(* Logix 5000 AddOnInstructionDefinition export Banner_Q20EAF_Param_v4; software revision 33.00 *)

TYPE Banner_IOL_Port_v4 :   // UDT that has all of the data items necessary to communicate with a specific Port on a IO-Link Master
STRUCT
   Port_Controlled : INT;   // Each bit represents a port on an IO-Link Master. Set to 1 to tell AOI to control that port.
   Port_Activate : INT;   // Each bit represents a port on an IO-Link Master. When ON that port will process any commands in queue.
   Port_Read : INT;   // Each bit represents a port on an IO-Link Master. Used to determine when device AOI has requested a Read command.
   Port_Write : INT;   // Each bit represents a port on an IO-Link Master. Used to determine when device AOI has requested a Write command.
   Port_RW_Complete : INT;   // Each bit represents a port on an IO-Link Master. Tells device AOI that Read or Write request has been completed.
   Port_Device_Read : INT;
   Data_Transfer : SINT[190];   // Array to transfer data from IO-Master to device AOIs.
END_STRUCT
END_TYPE

TYPE Banner_Q20EAF_RD_v4 :   // UDT that stores the Write Data for a Q20 EAF.
STRUCT
   Master_Cycle_Time : INT;
   Min_Cycle_Time : INT;
   M_Sequence_Capability : INT;
   IO_Link_Version_ID : INT;
   Process_Data_Input_Length : INT;
   Process_Data_Output_Length : INT;
   Combined_Vendor_ID : DINT;   // IO-Link Vendor ID
   Vendor_ID1 : INT;
   Vendor_ID2 : INT;
   Combined_Device_ID : DINT;   // IO-Link Device ID
   Device_ID1 : INT;
   Device_ID2 : INT;
   Device_ID3 : INT;
   Serial_Number : STRING;
   Teach_State : INT;   // 0 = Idle, 1 = SP1 Success, 4 = Wait for Command, 5 = Busy, 7 = Error.
   SP1_TP1 : SINT;
   SP1_TP2 : SINT;
   Current_Setpoint : DINT;   // Current setpoint selected by either the POT or SP1.
   All_Time_Run_Time : DINT;   // Read only counter that tracks the total time sensor has been running since manufacture. Value in Hours.
   Taught_Distance_Status : INT;   // 0 = Not taught, 1 = Taught, 2 = Coerced to near limit, 3 = Coerced to far limit.
END_STRUCT
END_TYPE

TYPE Banner_Q20EAF_v4 :   // All of the parameters for a Q20 EAF.
STRUCT
   Initial_Global_Read : BOOL;   // Determines if all of the IO-Link data has been read into the PLC yet
   Command : INT;   // Value placed in here will activate a read or write to a specifc IO-Link Index
   Read_Data : Banner_Q20EAF_RD_v4;   // Read Only Data
   Write_Data : Banner_Q20EAF_WD_v4;   // Write Data
   Archive : Banner_Q20EAF_WD_v4;   // Archive Data
   Reset : BOOL;   // Resets AOI. This will force a complete parameter read of the sensor.
END_STRUCT
END_TYPE

TYPE Banner_Q20EAF_WD_v4 :   // UDT that stores the Write Data for a Q20 EAF.
STRUCT
   System_Command : INT;   // See IODD file for list of commands that can be activated via the System Command interface
   Parameter_Access_Lock : SINT;   // Write access to all parameters is prohibited while value is 1. Only this parameter can be adjusted when value is 1.
   Data_Storage_Lock : SINT;   // Automatic data storage is disabled when this value is equal to 1. Read access is not affected.
   Local_Parameterization_Lock : SINT;   // Parameterization via local control elements on device is disabled.
   Local_User_Interface_Lock : SINT;   // Operation of local user interface is disabled.
   BDC1_Setpoint_SP1 : DINT;
   BDC1_Setpoint_SP2 : DINT;
   BDC1_Swithpoint_Logic : INT;   // 0 = Light Operate, 1 = Dark Operate
   BDC1_BDC_Mode : INT;   // 1 = 1-Pt BGS, 128 = 2-Pt, 129 = Dynamic, 130 = Window or FGS, 131 = Dual
   BDC1_Hysteresis : DINT;   // Should always be 0
   BDC1_Setpoint_Selection : SINT;   // 0 = Local (POT), 1 = Remote (AOI).
   Delay_Mode : INT;   // 0=Disabled, 1=On Off Delay, 2=Oneshot
   Delay_Timer_1 : DINT;   // 0 to 90000 ms
   Delay_Timer_2 : DINT;   // 0 to 90000 ms
   Teach_Offset_mode : INT;   // 0 = Auto, 1 = User Controlled.
   User_Teach_Offset : DINT;   // User selected teach offset.
   Resettable_Run_Time : DINT;
   All_Time_Run_Time_Event_Time : DINT;
   Resettable_Run_Time_Event_Time : DINT;
   Pin_2_Configuration : SINT;   // 0 = Detection Output, 1 = Complimentary Output.
   Response_Speed : SINT;   // 0 = High Speed (450 microsecs), 1 = Cross-talk Only (1.1 ms), 2 = Robust (1.7 ms ON, 1.1 ms OFF).
END_STRUCT
END_TYPE

ADD_ON_INSTRUCTION Banner_Q20EAF_Param_v4   (* revision 4.0, vendor Banner Engineering *)
// AOI to read and write parameter data to an IO-Link Q20 EAF.
VAR_IN_OUT
   Q20 : Banner_Q20EAF_v4; {required}
   Port_Data : Banner_IOL_Port_v4; {required}
END_VAR
VAR_INPUT
   Port : DINT; {required}
END_VAR
VAR
   Local_Control : DINT; {access None}
   Global_Read_Command_Value : INT; {access None}
   Global_Write_Command_Value : INT; {access None}
   Command_Being_Processed : BOOL; {access None}
   Update_Archive : BOOL; {access None}
   Index_Write_Inprocess : INT; {access None}
   Index_Write_Control : INT; {access None}
   Inprocess_Index : DINT; {access None}
END_VAR

ROUTINE Logic   (* ladder *)
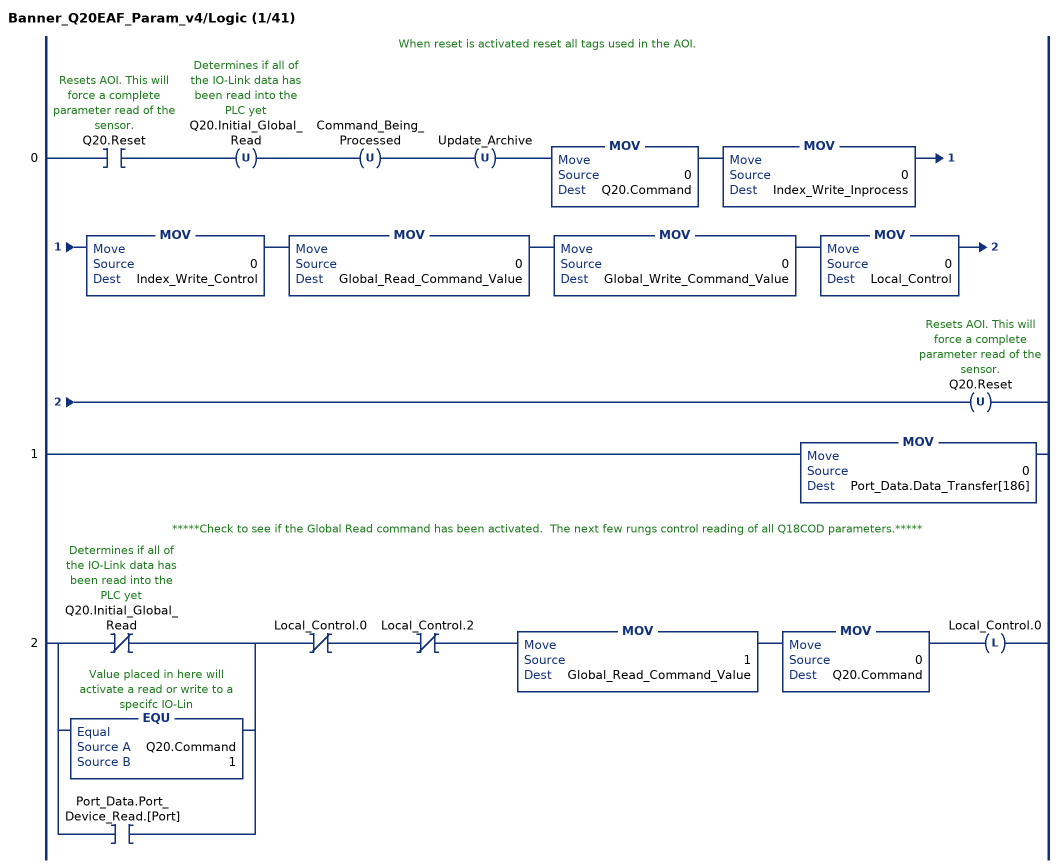
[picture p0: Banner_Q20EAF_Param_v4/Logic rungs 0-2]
   // When reset is activated reset all tags used in the AOI.
   0: XIC(Q20.Reset)OTU(Q20.Initial_Global_Read)OTU(Command_Being_Processed)OTU(Update_Archive)MOV(0,Q20.Command)MOV(0,Index_Write_Inprocess)MOV(0,Index_Write_Control)MOV(0,Global_Read_Command_Value)MOV(0,Global_Write_Command_Value)MOV(0,Local_Control)OTU(Q20.Reset);
   1: MOV(0,Port_Data.Data_Transfer[186]);
   // *****Check to see if the Global Read command has been activated.  The next few rungs control reading of all Q18COD parameters.*****
   2: [XIO(Q20.Initial_Global_Read) ,EQU(Q20.Command,1) ,XIC(Port_Data.Port_Device_Read.[Port]) ]XIO(Local_Control.0)XIO(Local_Control.2)MOV(1,Global_Read_Command_Value)MOV(0,Q20.Command)OTL(Local_Control.0);
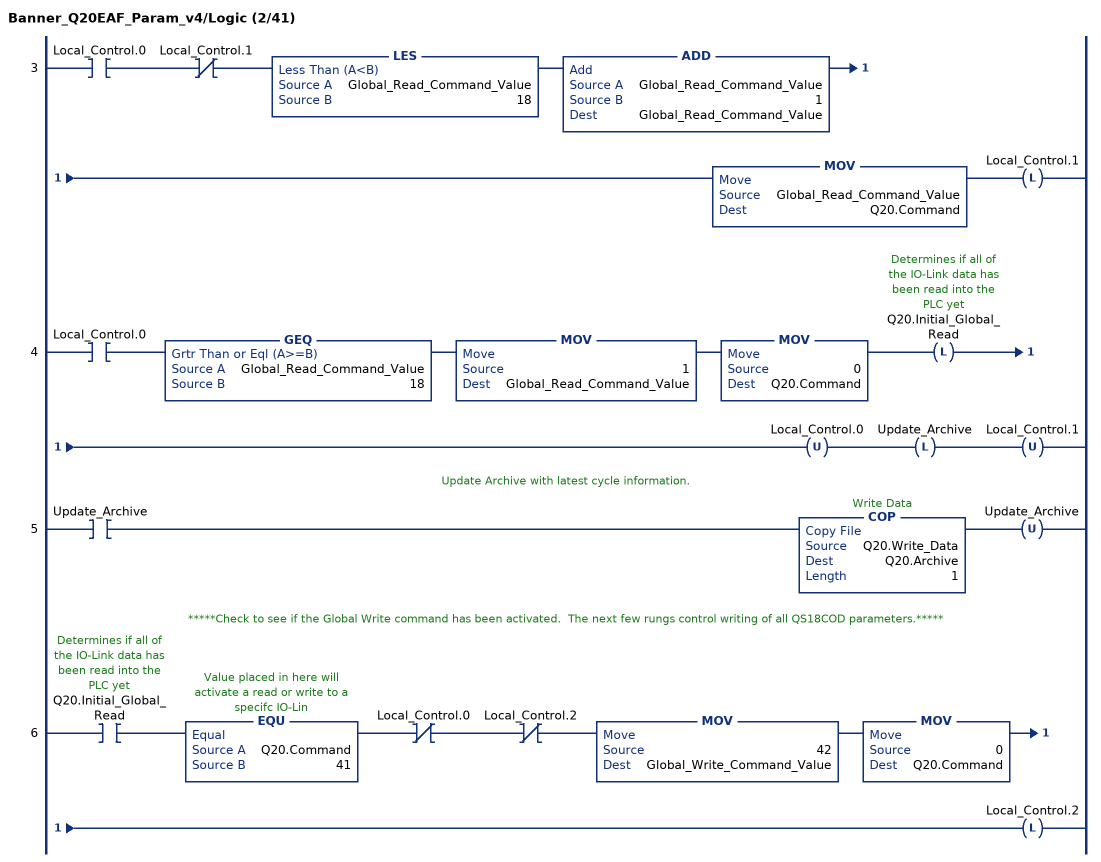
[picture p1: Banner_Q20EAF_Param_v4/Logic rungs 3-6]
   3: XIC(Local_Control.0)XIO(Local_Control.1)LES(Global_Read_Command_Value,18)ADD(Global_Read_Command_Value,1,Global_Read_Command_Value)MOV(Global_Read_Command_Value,Q20.Command)OTL(Local_Control.1);
   4: XIC(Local_Control.0)GEQ(Global_Read_Command_Value,18)MOV(1,Global_Read_Command_Value)MOV(0,Q20.Command)OTL(Q20.Initial_Global_Read)OTU(Local_Control.0)OTL(Update_Archive)OTU(Local_Control.1);
   // Update Archive with latest cycle information.
   5: XIC(Update_Archive)COP(Q20.Write_Data,Q20.Archive,1)OTU(Update_Archive);
   // *****Check to see if the Global Write command has been activated.  The next few rungs control writing of all QS18COD parameters.*****
   6: XIC(Q20.Initial_Global_Read)EQU(Q20.Command,41)XIO(Local_Control.0)XIO(Local_Control.2)MOV(42,Global_Write_Command_Value)MOV(0,Q20.Command)OTL(Local_Control.2);
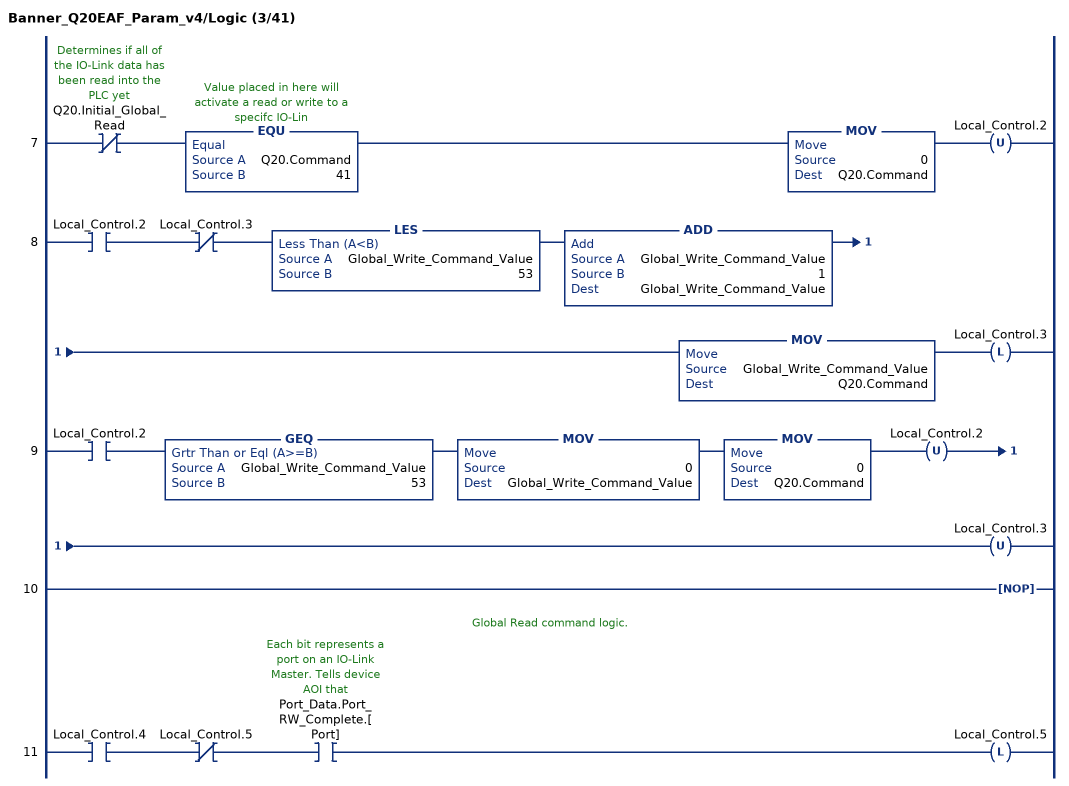
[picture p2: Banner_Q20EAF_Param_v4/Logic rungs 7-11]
   7: XIO(Q20.Initial_Global_Read)EQU(Q20.Command,41)MOV(0,Q20.Command)OTU(Local_Control.2);
   8: XIC(Local_Control.2)XIO(Local_Control.3)LES(Global_Write_Command_Value,53)ADD(Global_Write_Command_Value,1,Global_Write_Command_Value)MOV(Global_Write_Command_Value,Q20.Command)OTL(Local_Control.3);
   9: XIC(Local_Control.2)GEQ(Global_Write_Command_Value,53)MOV(0,Global_Write_Command_Value)MOV(0,Q20.Command)OTU(Local_Control.2)OTU(Local_Control.3);
   10: NOP();
   // Global Read command logic.
   11: XIC(Local_Control.4)XIO(Local_Control.5)XIC(Port_Data.Port_RW_Complete.[Port])OTL(Local_Control.5);
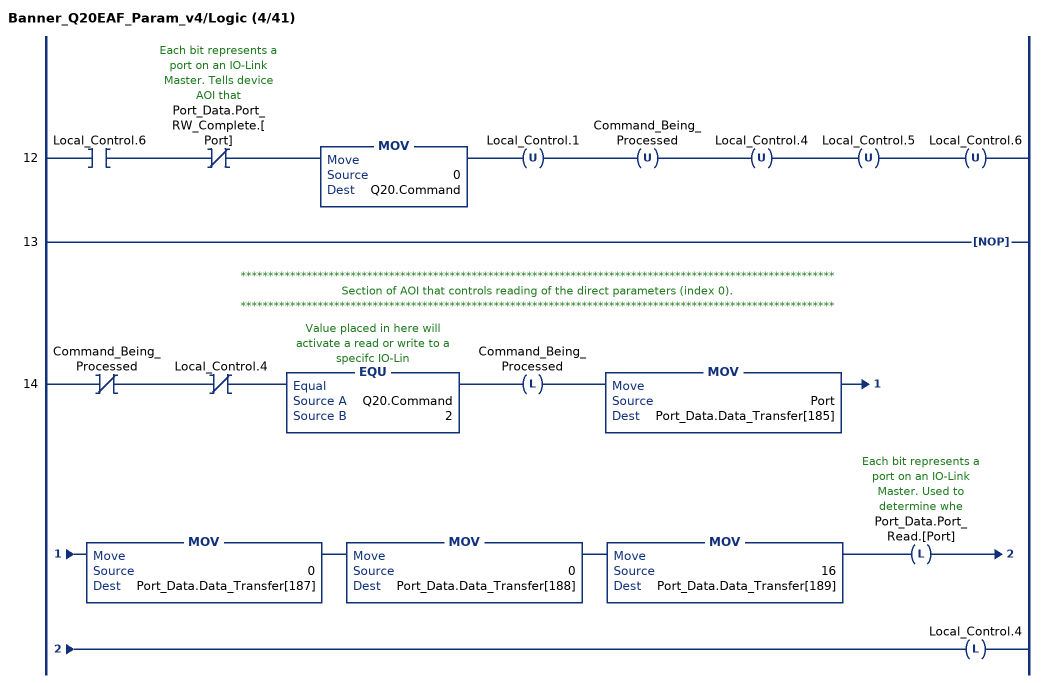
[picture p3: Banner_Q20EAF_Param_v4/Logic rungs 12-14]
   12: XIC(Local_Control.6)XIO(Port_Data.Port_RW_Complete.[Port])MOV(0,Q20.Command)OTU(Local_Control.1)OTU(Command_Being_Processed)OTU(Local_Control.4)OTU(Local_Control.5)OTU(Local_Control.6);
   13: NOP();
   // ************************************************************************************************************
   // Section of AOI that controls reading of the direct parameters (index 0).
   // ************************************************************************************************************
   14: XIO(Command_Being_Processed)XIO(Local_Control.4)EQU(Q20.Command,2)OTL(Command_Being_Processed)MOV(Port,Port_Data.Data_Transfer[185])MOV(0,Port_Data.Data_Transfer[187])MOV(0,Port_Data.Data_Transfer[188])MOV(16,Port_Data.Data_Transfer[189])OTL(Port_Data.Port_Read.[Port])OTL(Local_Control.4);
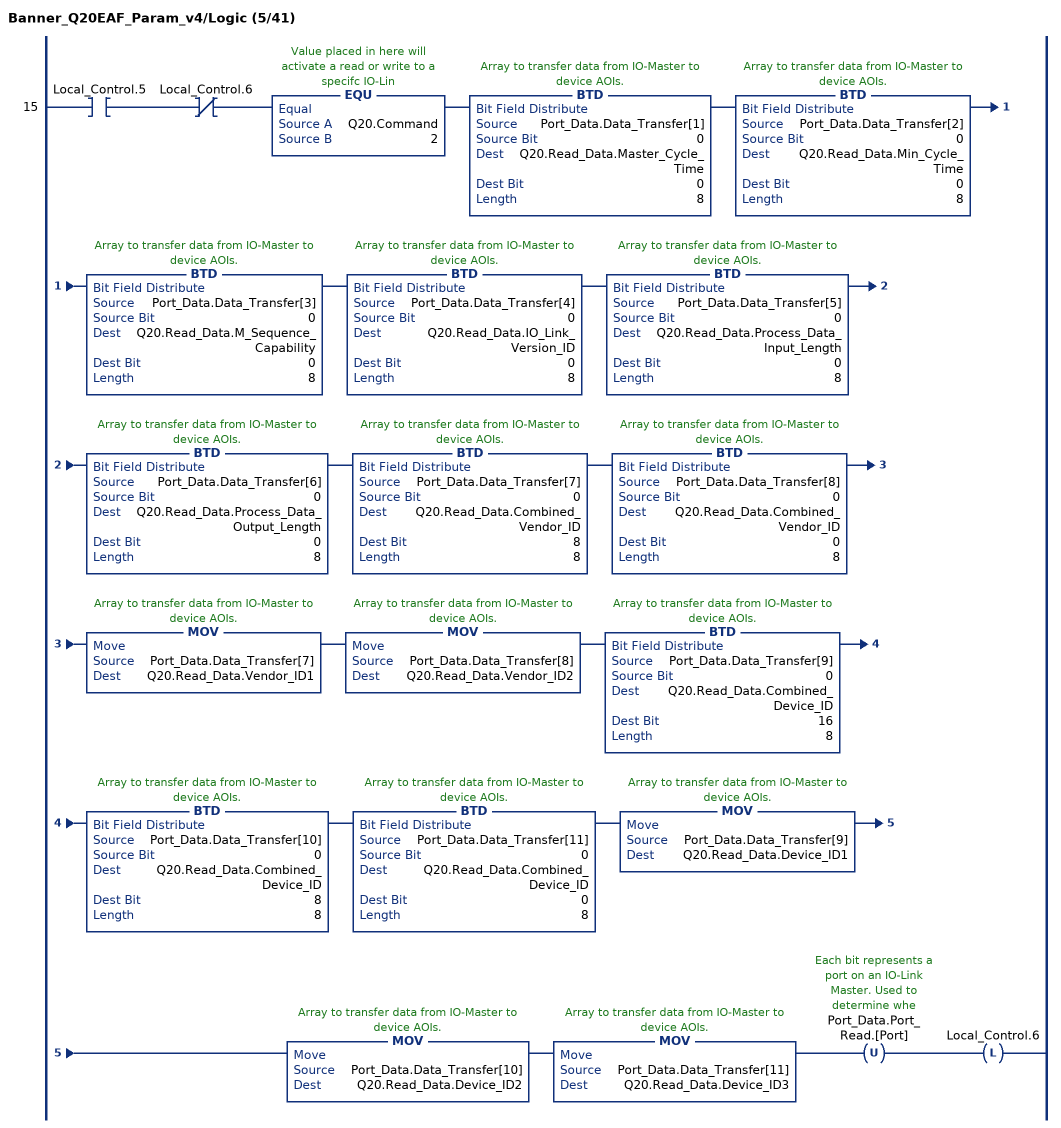
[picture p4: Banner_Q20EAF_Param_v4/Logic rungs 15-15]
   15: XIC(Local_Control.5)XIO(Local_Control.6)EQU(Q20.Command,2)BTD(Port_Data.Data_Transfer[1],0,Q20.Read_Data.Master_Cycle_Time,0,8)BTD(Port_Data.Data_Transfer[2],0,Q20.Read_Data.Min_Cycle_Time,0,8)BTD(Port_Data.Data_Transfer[3],0,Q20.Read_Data.M_Sequence_Capability,0,8)BTD(Port_Data.Data_Transfer[4],0,Q20.Read_Data.IO_Link_Version_ID,0,8)BTD(Port_Data.Data_Transfer[5],0,Q20.Read_Data.Process_Data_Input_Length,0,8)BTD(Port_Data.Data_Transfer[6],0,Q20.Read_Data.Process_Data_Output_Length,0,8)BTD(Port_Data.Data_Transfer[7],0,Q20.Read_Data.Combined_Vendor_ID,8,8)BTD(Port_Data.Data_Transfer[8],0,Q20.Read_Data.Combined_Vendor_ID,0,8)MOV(Port_Data.Data_Transfer[7],Q20.Read_Data.Vendor_ID1)MOV(Port_Data.Data_Transfer[8],Q20.Read_Data.Vendor_ID2)BTD(Port_Data.Data_Transfer[9],0,Q20.Read_Data.Combined_Device_ID,16,8)BTD(Port_Data.Data_Transfer[10],0,Q20.Read_Data.Combined_Device_ID,8,8)BTD(Port_Data.Data_Transfer[11],0,Q20.Read_Data.Combined_Device_ID,0,8)MOV(Port_Data.Data_Transfer[9],Q20.Read_Data.Device_ID1)MOV(Port_Data.Data_Transfer[10],Q20.Read_Data.Device_ID2)MOV(Port_Data.Data_Transfer[11],Q20.Read_Data.Device_ID3)OTU(Port_Data.Port_Read.[Port])OTL(Local_Control.6);
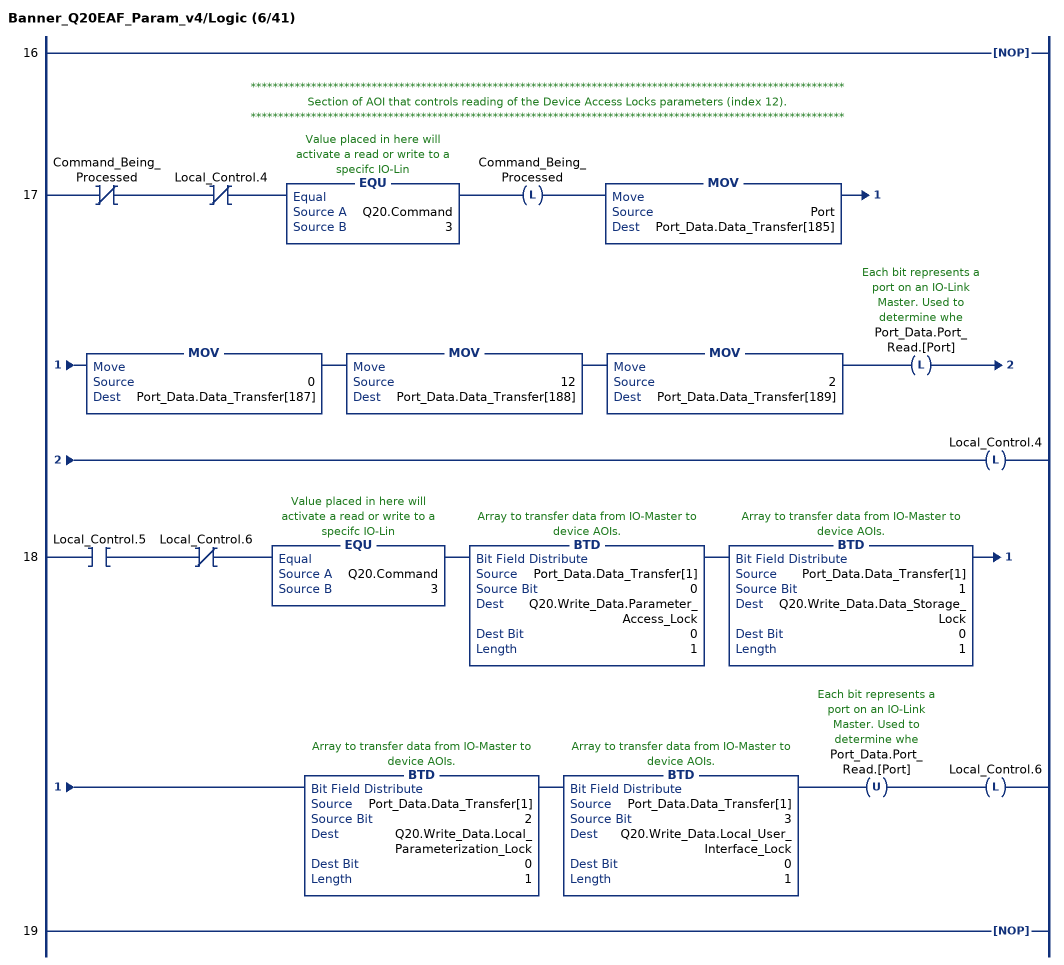
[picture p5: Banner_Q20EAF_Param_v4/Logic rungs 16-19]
   16: NOP();
   // ************************************************************************************************************
   // Section of AOI that controls reading of the Device Access Locks parameters (index 12).
   // ************************************************************************************************************
   17: XIO(Command_Being_Processed)XIO(Local_Control.4)EQU(Q20.Command,3)OTL(Command_Being_Processed)MOV(Port,Port_Data.Data_Transfer[185])MOV(0,Port_Data.Data_Transfer[187])MOV(12,Port_Data.Data_Transfer[188])MOV(2,Port_Data.Data_Transfer[189])OTL(Port_Data.Port_Read.[Port])OTL(Local_Control.4);
   18: XIC(Local_Control.5)XIO(Local_Control.6)EQU(Q20.Command,3)BTD(Port_Data.Data_Transfer[1],0,Q20.Write_Data.Parameter_Access_Lock,0,1)BTD(Port_Data.Data_Transfer[1],1,Q20.Write_Data.Data_Storage_Lock,0,1)BTD(Port_Data.Data_Transfer[1],2,Q20.Write_Data.Local_Parameterization_Lock,0,1)BTD(Port_Data.Data_Transfer[1],3,Q20.Write_Data.Local_User_Interface_Lock,0,1)OTU(Port_Data.Port_Read.[Port])OTL(Local_Control.6);
   19: NOP();
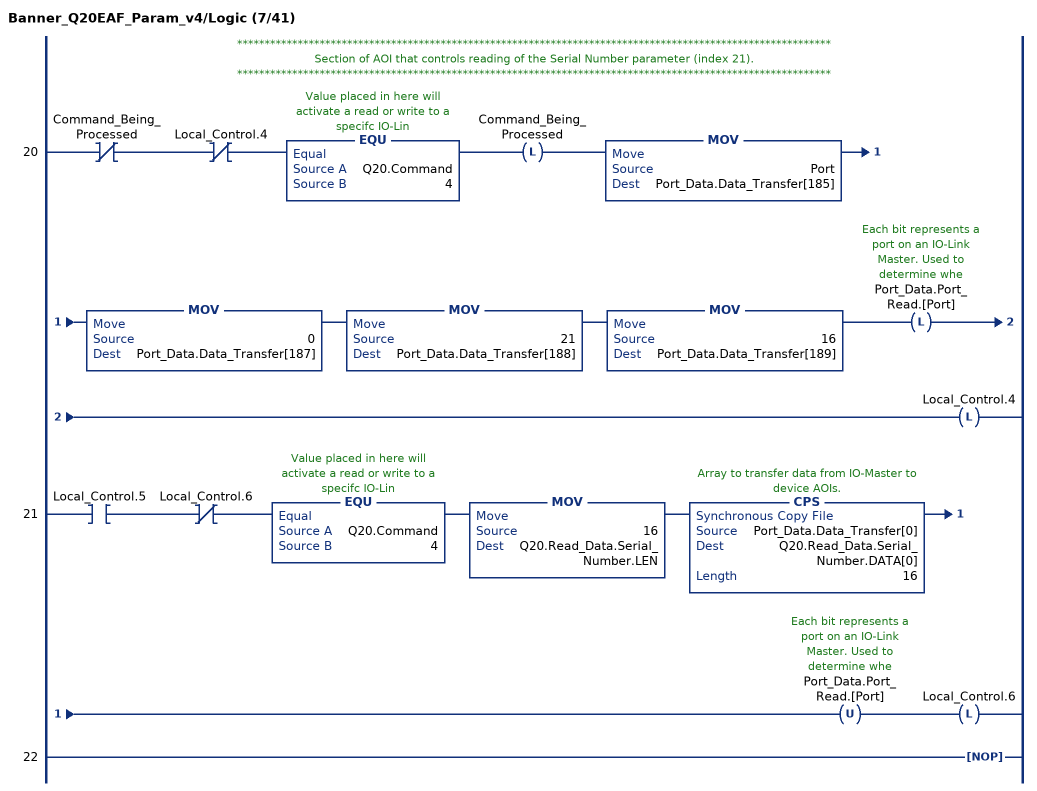
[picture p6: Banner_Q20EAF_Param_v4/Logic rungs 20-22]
   // ************************************************************************************************************
   // Section of AOI that controls reading of the Serial Number parameter (index 21).
   // ************************************************************************************************************
   20: XIO(Command_Being_Processed)XIO(Local_Control.4)EQU(Q20.Command,4)OTL(Command_Being_Processed)MOV(Port,Port_Data.Data_Transfer[185])MOV(0,Port_Data.Data_Transfer[187])MOV(21,Port_Data.Data_Transfer[188])MOV(16,Port_Data.Data_Transfer[189])OTL(Port_Data.Port_Read.[Port])OTL(Local_Control.4);
   21: XIC(Local_Control.5)XIO(Local_Control.6)EQU(Q20.Command,4)MOV(16,Q20.Read_Data.Serial_Number.LEN)CPS(Port_Data.Data_Transfer[0],Q20.Read_Data.Serial_Number.DATA[0],16)OTU(Port_Data.Port_Read.[Port])OTL(Local_Control.6);
   22: NOP();
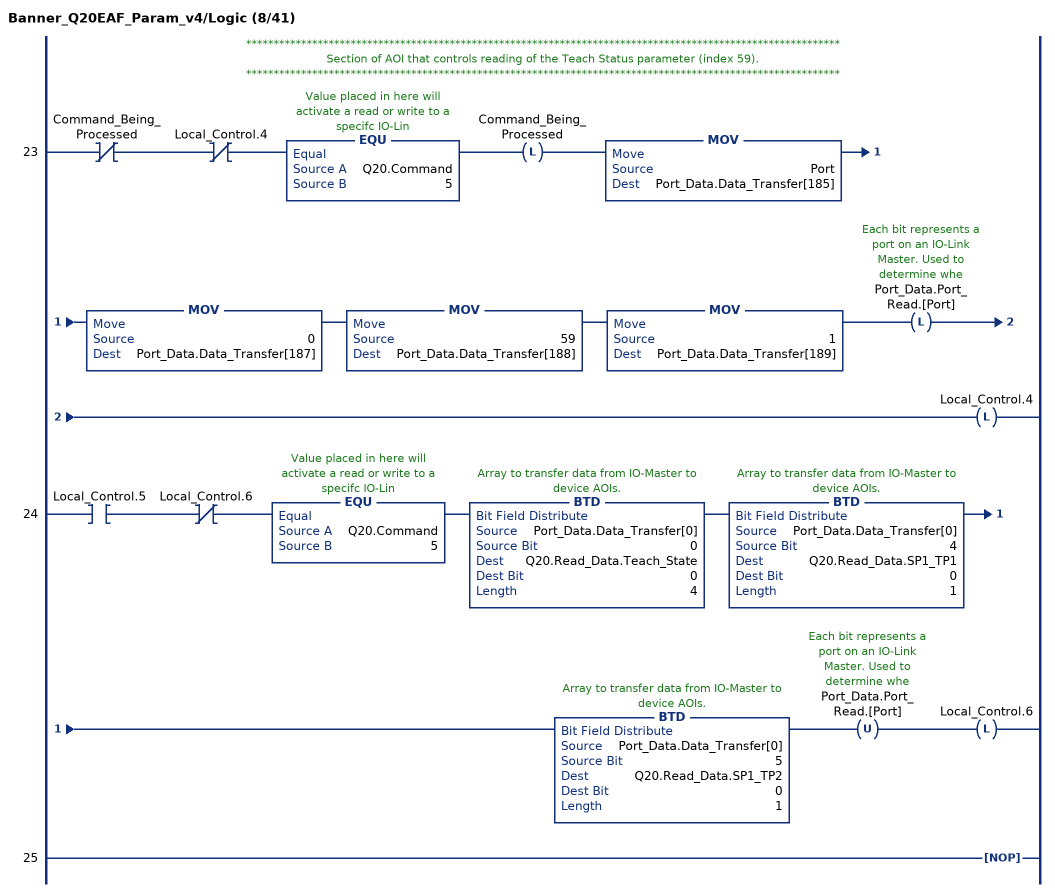
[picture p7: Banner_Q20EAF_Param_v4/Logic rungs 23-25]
   // ************************************************************************************************************
   // Section of AOI that controls reading of the Teach Status parameter (index 59).
   // ************************************************************************************************************
   23: XIO(Command_Being_Processed)XIO(Local_Control.4)EQU(Q20.Command,5)OTL(Command_Being_Processed)MOV(Port,Port_Data.Data_Transfer[185])MOV(0,Port_Data.Data_Transfer[187])MOV(59,Port_Data.Data_Transfer[188])MOV(1,Port_Data.Data_Transfer[189])OTL(Port_Data.Port_Read.[Port])OTL(Local_Control.4);
   24: XIC(Local_Control.5)XIO(Local_Control.6)EQU(Q20.Command,5)BTD(Port_Data.Data_Transfer[0],0,Q20.Read_Data.Teach_State,0,4)BTD(Port_Data.Data_Transfer[0],4,Q20.Read_Data.SP1_TP1,0,1)BTD(Port_Data.Data_Transfer[0],5,Q20.Read_Data.SP1_TP2,0,1)OTU(Port_Data.Port_Read.[Port])OTL(Local_Control.6);
   25: NOP();
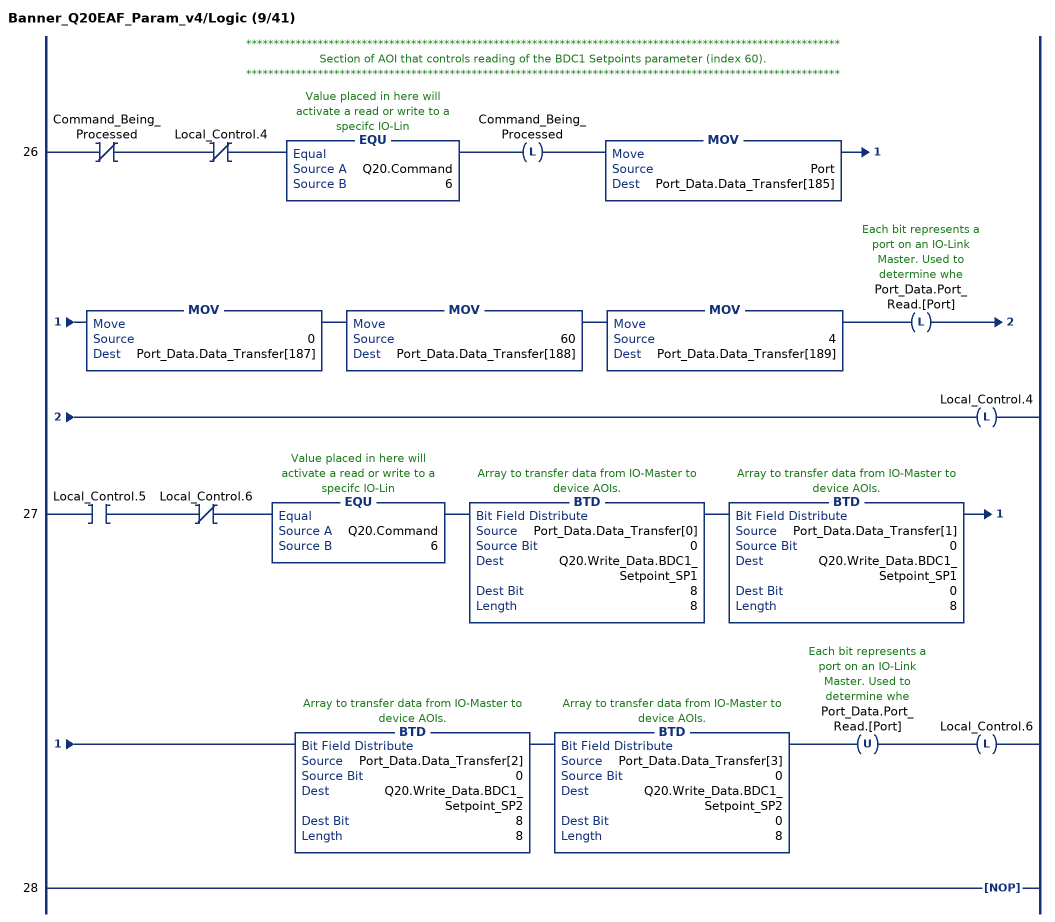
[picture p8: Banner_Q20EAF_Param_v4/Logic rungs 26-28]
   // ************************************************************************************************************
   // Section of AOI that controls reading of the BDC1 Setpoints parameter (index 60).
   // ************************************************************************************************************
   26: XIO(Command_Being_Processed)XIO(Local_Control.4)EQU(Q20.Command,6)OTL(Command_Being_Processed)MOV(Port,Port_Data.Data_Transfer[185])MOV(0,Port_Data.Data_Transfer[187])MOV(60,Port_Data.Data_Transfer[188])MOV(4,Port_Data.Data_Transfer[189])OTL(Port_Data.Port_Read.[Port])OTL(Local_Control.4);
   27: XIC(Local_Control.5)XIO(Local_Control.6)EQU(Q20.Command,6)BTD(Port_Data.Data_Transfer[0],0,Q20.Write_Data.BDC1_Setpoint_SP1,8,8)BTD(Port_Data.Data_Transfer[1],0,Q20.Write_Data.BDC1_Setpoint_SP1,0,8)BTD(Port_Data.Data_Transfer[2],0,Q20.Write_Data.BDC1_Setpoint_SP2,8,8)BTD(Port_Data.Data_Transfer[3],0,Q20.Write_Data.BDC1_Setpoint_SP2,0,8)OTU(Port_Data.Port_Read.[Port])OTL(Local_Control.6);
   28: NOP();
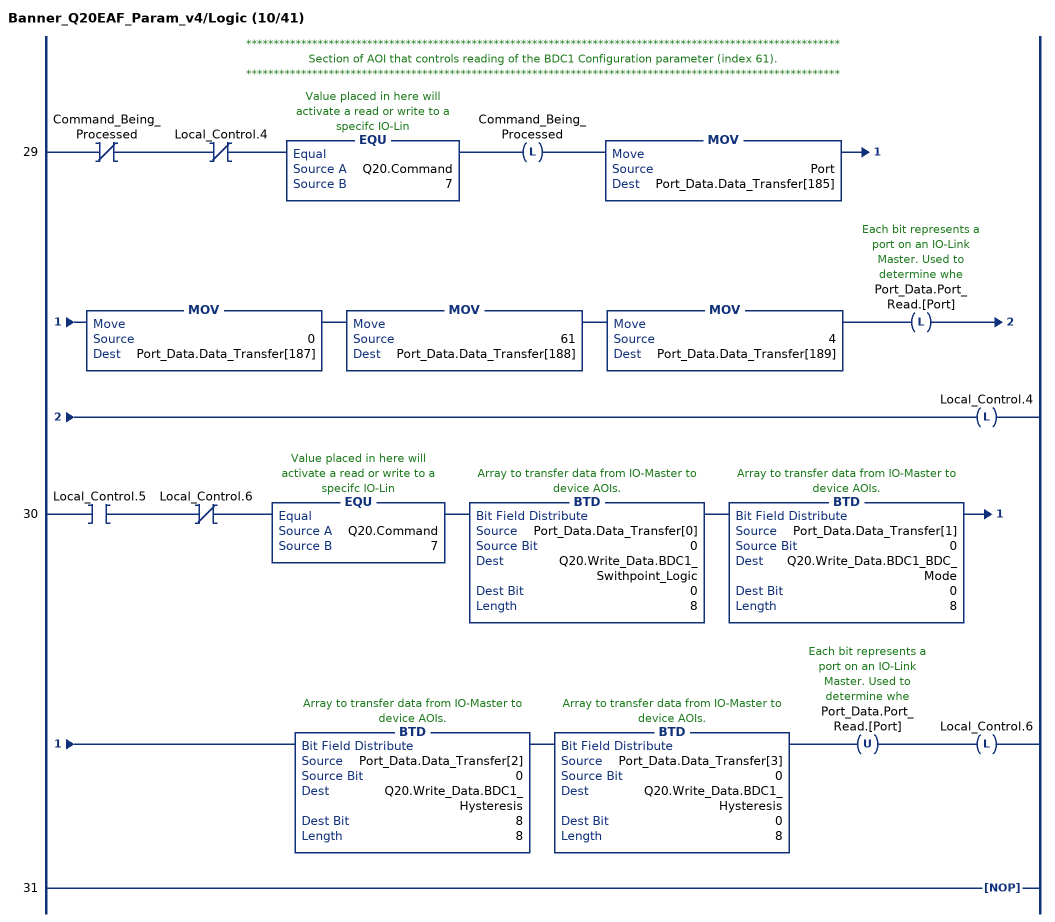
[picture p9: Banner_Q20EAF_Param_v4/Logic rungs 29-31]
   // ************************************************************************************************************
   // Section of AOI that controls reading of the BDC1 Configuration parameter (index 61).
   // ************************************************************************************************************
   29: XIO(Command_Being_Processed)XIO(Local_Control.4)EQU(Q20.Command,7)OTL(Command_Being_Processed)MOV(Port,Port_Data.Data_Transfer[185])MOV(0,Port_Data.Data_Transfer[187])MOV(61,Port_Data.Data_Transfer[188])MOV(4,Port_Data.Data_Transfer[189])OTL(Port_Data.Port_Read.[Port])OTL(Local_Control.4);
   30: XIC(Local_Control.5)XIO(Local_Control.6)EQU(Q20.Command,7)BTD(Port_Data.Data_Transfer[0],0,Q20.Write_Data.BDC1_Swithpoint_Logic,0,8)BTD(Port_Data.Data_Transfer[1],0,Q20.Write_Data.BDC1_BDC_Mode,0,8)BTD(Port_Data.Data_Transfer[2],0,Q20.Write_Data.BDC1_Hysteresis,8,8)BTD(Port_Data.Data_Transfer[3],0,Q20.Write_Data.BDC1_Hysteresis,0,8)OTU(Port_Data.Port_Read.[Port])OTL(Local_Control.6);
   31: NOP();
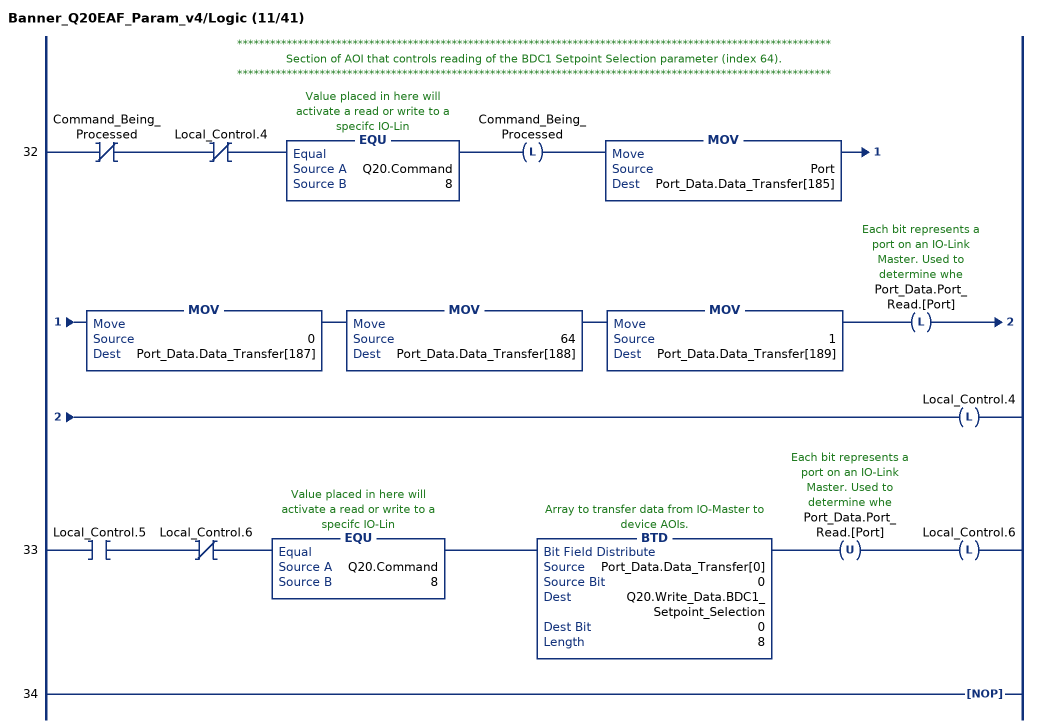
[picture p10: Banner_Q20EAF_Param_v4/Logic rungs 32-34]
   // ************************************************************************************************************
   // Section of AOI that controls reading of the BDC1 Setpoint Selection parameter (index 64).
   // ************************************************************************************************************
   32: XIO(Command_Being_Processed)XIO(Local_Control.4)EQU(Q20.Command,8)OTL(Command_Being_Processed)MOV(Port,Port_Data.Data_Transfer[185])MOV(0,Port_Data.Data_Transfer[187])MOV(64,Port_Data.Data_Transfer[188])MOV(1,Port_Data.Data_Transfer[189])OTL(Port_Data.Port_Read.[Port])OTL(Local_Control.4);
   33: XIC(Local_Control.5)XIO(Local_Control.6)EQU(Q20.Command,8)BTD(Port_Data.Data_Transfer[0],0,Q20.Write_Data.BDC1_Setpoint_Selection,0,8)OTU(Port_Data.Port_Read.[Port])OTL(Local_Control.6);
   34: NOP();
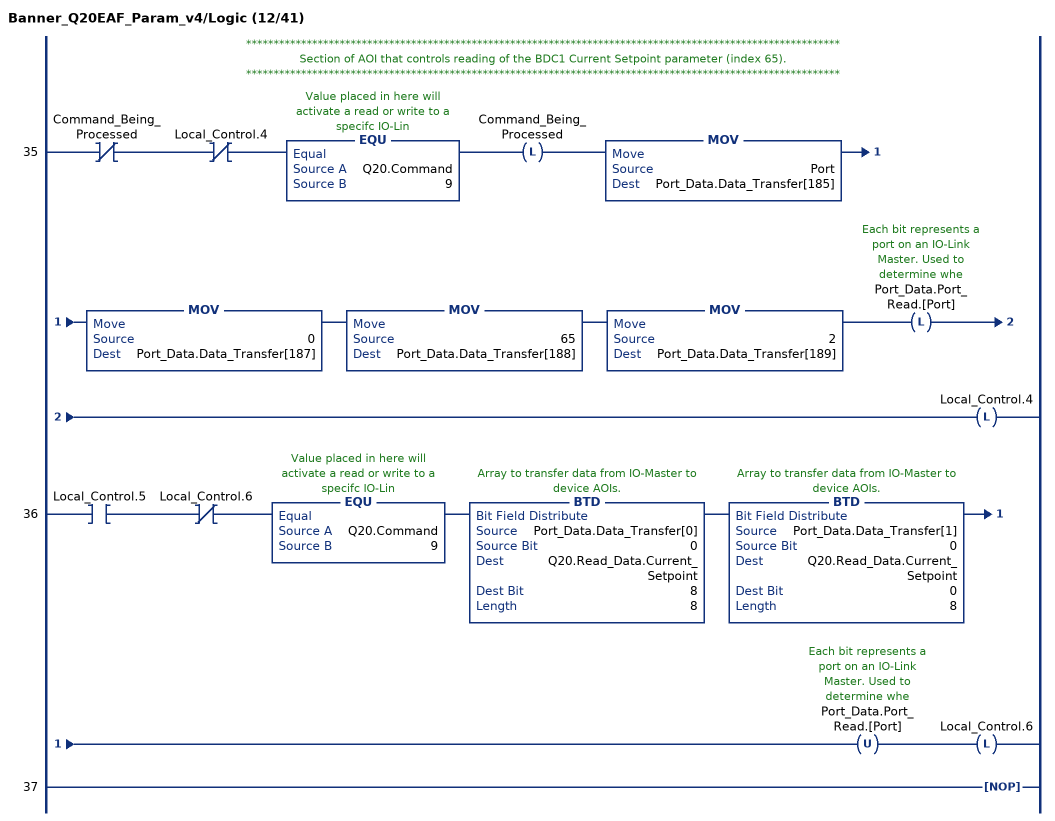
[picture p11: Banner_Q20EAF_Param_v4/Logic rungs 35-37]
   // ************************************************************************************************************
   // Section of AOI that controls reading of the BDC1 Current Setpoint parameter (index 65).
   // ************************************************************************************************************
   35: XIO(Command_Being_Processed)XIO(Local_Control.4)EQU(Q20.Command,9)OTL(Command_Being_Processed)MOV(Port,Port_Data.Data_Transfer[185])MOV(0,Port_Data.Data_Transfer[187])MOV(65,Port_Data.Data_Transfer[188])MOV(2,Port_Data.Data_Transfer[189])OTL(Port_Data.Port_Read.[Port])OTL(Local_Control.4);
   36: XIC(Local_Control.5)XIO(Local_Control.6)EQU(Q20.Command,9)BTD(Port_Data.Data_Transfer[0],0,Q20.Read_Data.Current_Setpoint,8,8)BTD(Port_Data.Data_Transfer[1],0,Q20.Read_Data.Current_Setpoint,0,8)OTU(Port_Data.Port_Read.[Port])OTL(Local_Control.6);
   37: NOP();
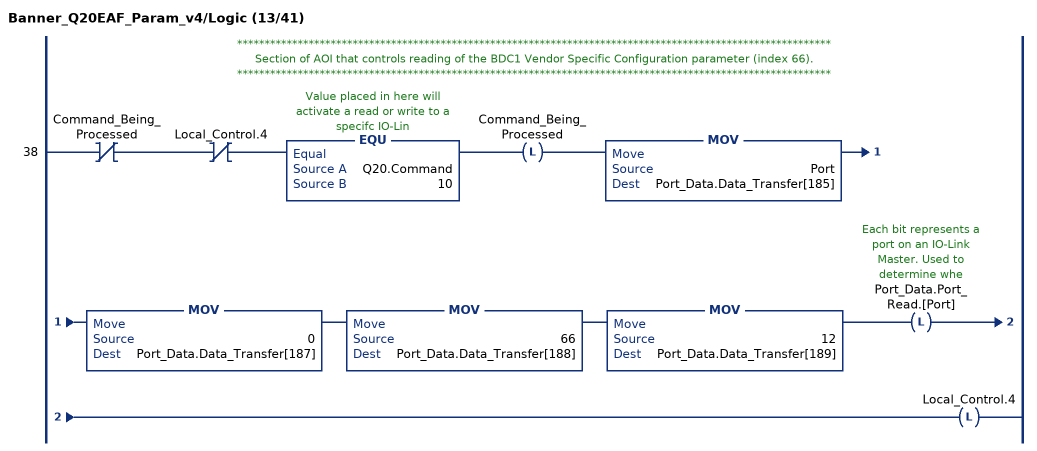
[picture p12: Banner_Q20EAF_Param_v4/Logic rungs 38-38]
   // ************************************************************************************************************
   // Section of AOI that controls reading of the BDC1 Vendor Specific Configuration parameter (index 66).
   // ************************************************************************************************************
   38: XIO(Command_Being_Processed)XIO(Local_Control.4)EQU(Q20.Command,10)OTL(Command_Being_Processed)MOV(Port,Port_Data.Data_Transfer[185])MOV(0,Port_Data.Data_Transfer[187])MOV(66,Port_Data.Data_Transfer[188])MOV(12,Port_Data.Data_Transfer[189])OTL(Port_Data.Port_Read.[Port])OTL(Local_Control.4);
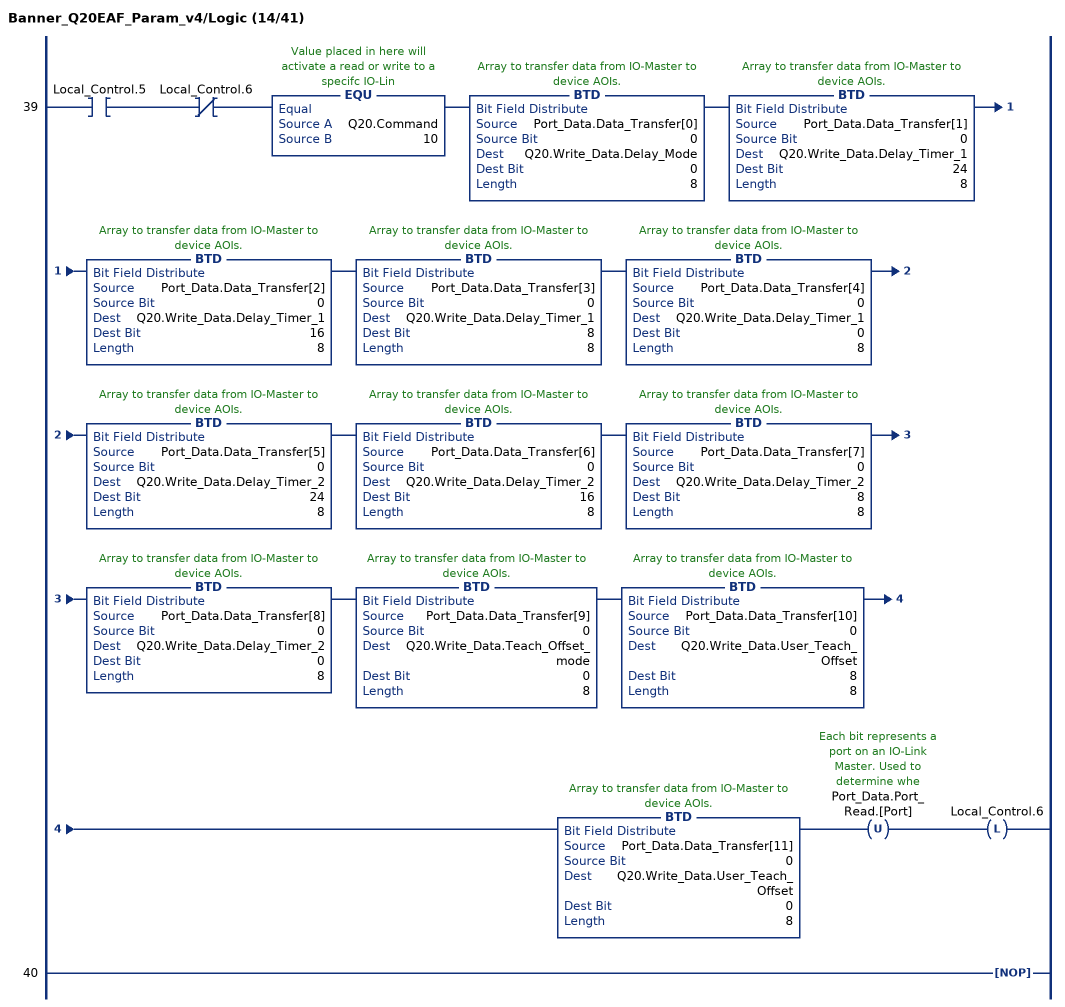
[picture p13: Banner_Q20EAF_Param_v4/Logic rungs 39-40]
   39: XIC(Local_Control.5)XIO(Local_Control.6)EQU(Q20.Command,10)BTD(Port_Data.Data_Transfer[0],0,Q20.Write_Data.Delay_Mode,0,8)BTD(Port_Data.Data_Transfer[1],0,Q20.Write_Data.Delay_Timer_1,24,8)BTD(Port_Data.Data_Transfer[2],0,Q20.Write_Data.Delay_Timer_1,16,8)BTD(Port_Data.Data_Transfer[3],0,Q20.Write_Data.Delay_Timer_1,8,8)BTD(Port_Data.Data_Transfer[4],0,Q20.Write_Data.Delay_Timer_1,0,8)BTD(Port_Data.Data_Transfer[5],0,Q20.Write_Data.Delay_Timer_2,24,8)BTD(Port_Data.Data_Transfer[6],0,Q20.Write_Data.Delay_Timer_2,16,8)BTD(Port_Data.Data_Transfer[7],0,Q20.Write_Data.Delay_Timer_2,8,8)BTD(Port_Data.Data_Transfer[8],0,Q20.Write_Data.Delay_Timer_2,0,8)BTD(Port_Data.Data_Transfer[9],0,Q20.Write_Data.Teach_Offset_mode,0,8)BTD(Port_Data.Data_Transfer[10],0,Q20.Write_Data.User_Teach_Offset,8,8)BTD(Port_Data.Data_Transfer[11],0,Q20.Write_Data.User_Teach_Offset,0,8)OTU(Port_Data.Port_Read.[Port])OTL(Local_Control.6);
   40: NOP();
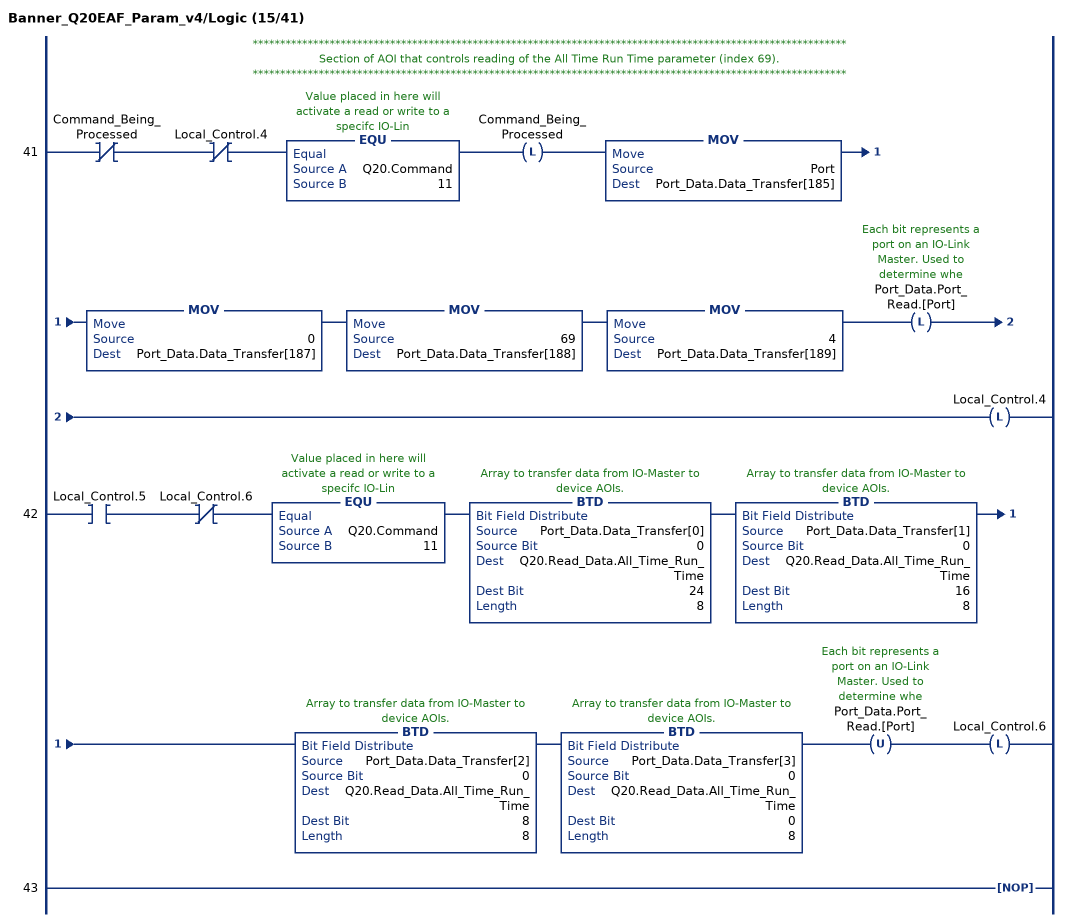
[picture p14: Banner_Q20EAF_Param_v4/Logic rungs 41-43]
   // ************************************************************************************************************
   // Section of AOI that controls reading of the All Time Run Time parameter (index 69).
   // ************************************************************************************************************
   41: XIO(Command_Being_Processed)XIO(Local_Control.4)EQU(Q20.Command,11)OTL(Command_Being_Processed)MOV(Port,Port_Data.Data_Transfer[185])MOV(0,Port_Data.Data_Transfer[187])MOV(69,Port_Data.Data_Transfer[188])MOV(4,Port_Data.Data_Transfer[189])OTL(Port_Data.Port_Read.[Port])OTL(Local_Control.4);
   42: XIC(Local_Control.5)XIO(Local_Control.6)EQU(Q20.Command,11)BTD(Port_Data.Data_Transfer[0],0,Q20.Read_Data.All_Time_Run_Time,24,8)BTD(Port_Data.Data_Transfer[1],0,Q20.Read_Data.All_Time_Run_Time,16,8)BTD(Port_Data.Data_Transfer[2],0,Q20.Read_Data.All_Time_Run_Time,8,8)BTD(Port_Data.Data_Transfer[3],0,Q20.Read_Data.All_Time_Run_Time,0,8)OTU(Port_Data.Port_Read.[Port])OTL(Local_Control.6);
   43: NOP();
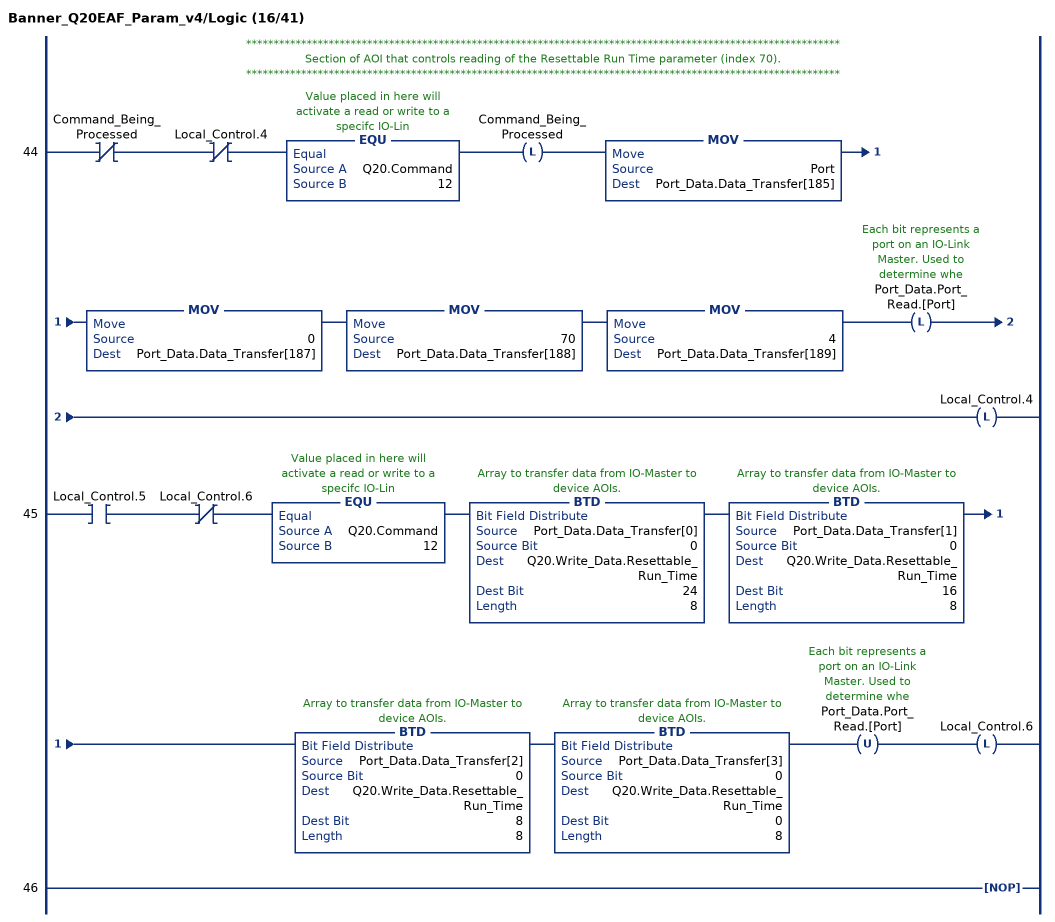
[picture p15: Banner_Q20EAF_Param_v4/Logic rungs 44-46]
   // ************************************************************************************************************
   // Section of AOI that controls reading of the Resettable Run Time parameter (index 70).
   // ************************************************************************************************************
   44: XIO(Command_Being_Processed)XIO(Local_Control.4)EQU(Q20.Command,12)OTL(Command_Being_Processed)MOV(Port,Port_Data.Data_Transfer[185])MOV(0,Port_Data.Data_Transfer[187])MOV(70,Port_Data.Data_Transfer[188])MOV(4,Port_Data.Data_Transfer[189])OTL(Port_Data.Port_Read.[Port])OTL(Local_Control.4);
   45: XIC(Local_Control.5)XIO(Local_Control.6)EQU(Q20.Command,12)BTD(Port_Data.Data_Transfer[0],0,Q20.Write_Data.Resettable_Run_Time,24,8)BTD(Port_Data.Data_Transfer[1],0,Q20.Write_Data.Resettable_Run_Time,16,8)BTD(Port_Data.Data_Transfer[2],0,Q20.Write_Data.Resettable_Run_Time,8,8)BTD(Port_Data.Data_Transfer[3],0,Q20.Write_Data.Resettable_Run_Time,0,8)OTU(Port_Data.Port_Read.[Port])OTL(Local_Control.6);
   46: NOP();
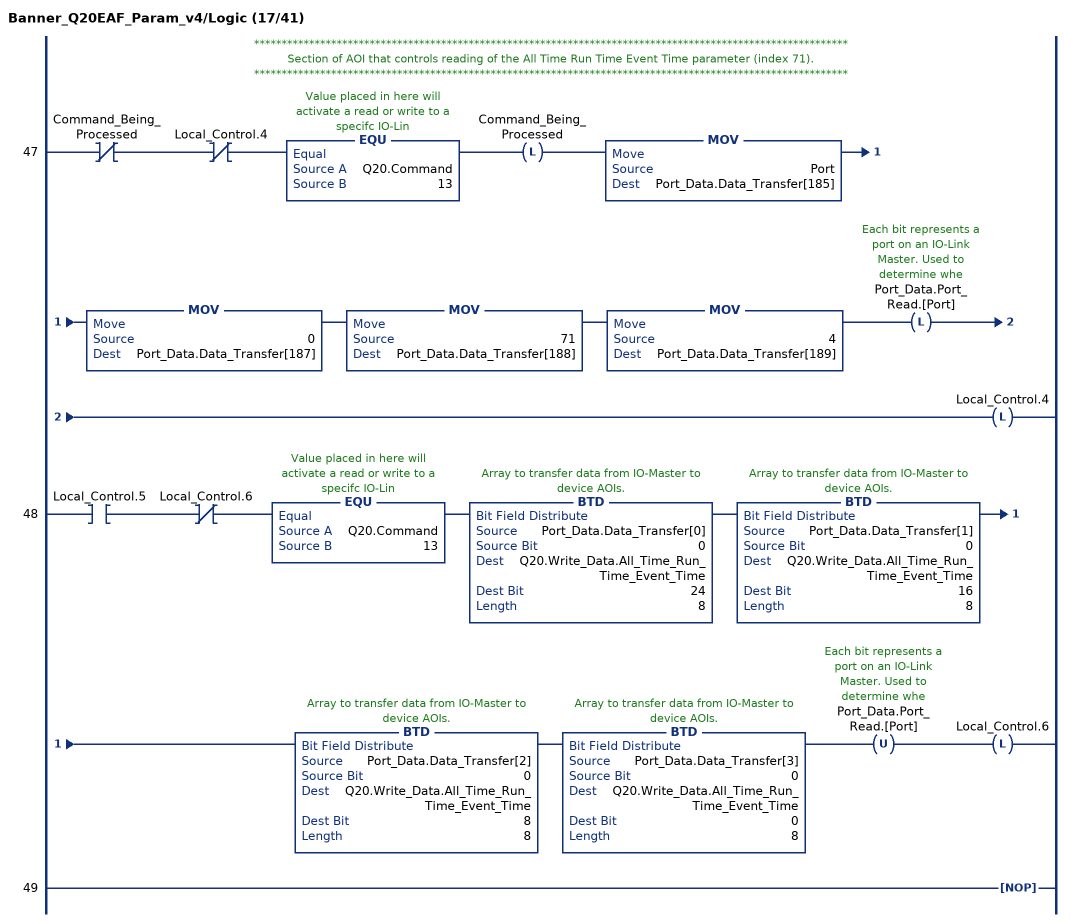
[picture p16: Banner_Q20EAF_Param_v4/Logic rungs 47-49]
   // ************************************************************************************************************
   // Section of AOI that controls reading of the All Time Run Time Event Time parameter (index 71).
   // ************************************************************************************************************
   47: XIO(Command_Being_Processed)XIO(Local_Control.4)EQU(Q20.Command,13)OTL(Command_Being_Processed)MOV(Port,Port_Data.Data_Transfer[185])MOV(0,Port_Data.Data_Transfer[187])MOV(71,Port_Data.Data_Transfer[188])MOV(4,Port_Data.Data_Transfer[189])OTL(Port_Data.Port_Read.[Port])OTL(Local_Control.4);
   48: XIC(Local_Control.5)XIO(Local_Control.6)EQU(Q20.Command,13)BTD(Port_Data.Data_Transfer[0],0,Q20.Write_Data.All_Time_Run_Time_Event_Time,24,8)BTD(Port_Data.Data_Transfer[1],0,Q20.Write_Data.All_Time_Run_Time_Event_Time,16,8)BTD(Port_Data.Data_Transfer[2],0,Q20.Write_Data.All_Time_Run_Time_Event_Time,8,8)BTD(Port_Data.Data_Transfer[3],0,Q20.Write_Data.All_Time_Run_Time_Event_Time,0,8)OTU(Port_Data.Port_Read.[Port])OTL(Local_Control.6);
   49: NOP();
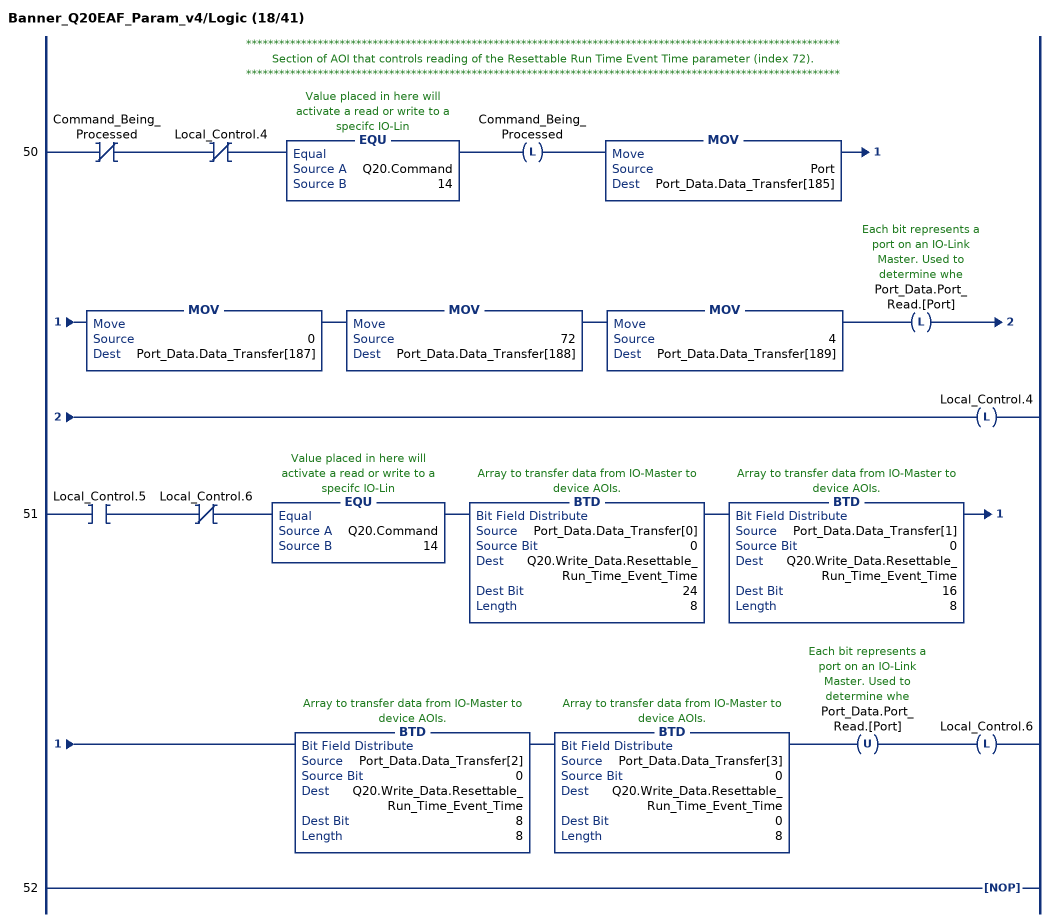
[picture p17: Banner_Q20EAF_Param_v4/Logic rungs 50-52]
   // ************************************************************************************************************
   // Section of AOI that controls reading of the Resettable Run Time Event Time parameter (index 72).
   // ************************************************************************************************************
   50: XIO(Command_Being_Processed)XIO(Local_Control.4)EQU(Q20.Command,14)OTL(Command_Being_Processed)MOV(Port,Port_Data.Data_Transfer[185])MOV(0,Port_Data.Data_Transfer[187])MOV(72,Port_Data.Data_Transfer[188])MOV(4,Port_Data.Data_Transfer[189])OTL(Port_Data.Port_Read.[Port])OTL(Local_Control.4);
   51: XIC(Local_Control.5)XIO(Local_Control.6)EQU(Q20.Command,14)BTD(Port_Data.Data_Transfer[0],0,Q20.Write_Data.Resettable_Run_Time_Event_Time,24,8)BTD(Port_Data.Data_Transfer[1],0,Q20.Write_Data.Resettable_Run_Time_Event_Time,16,8)BTD(Port_Data.Data_Transfer[2],0,Q20.Write_Data.Resettable_Run_Time_Event_Time,8,8)BTD(Port_Data.Data_Transfer[3],0,Q20.Write_Data.Resettable_Run_Time_Event_Time,0,8)OTU(Port_Data.Port_Read.[Port])OTL(Local_Control.6);
   52: NOP();
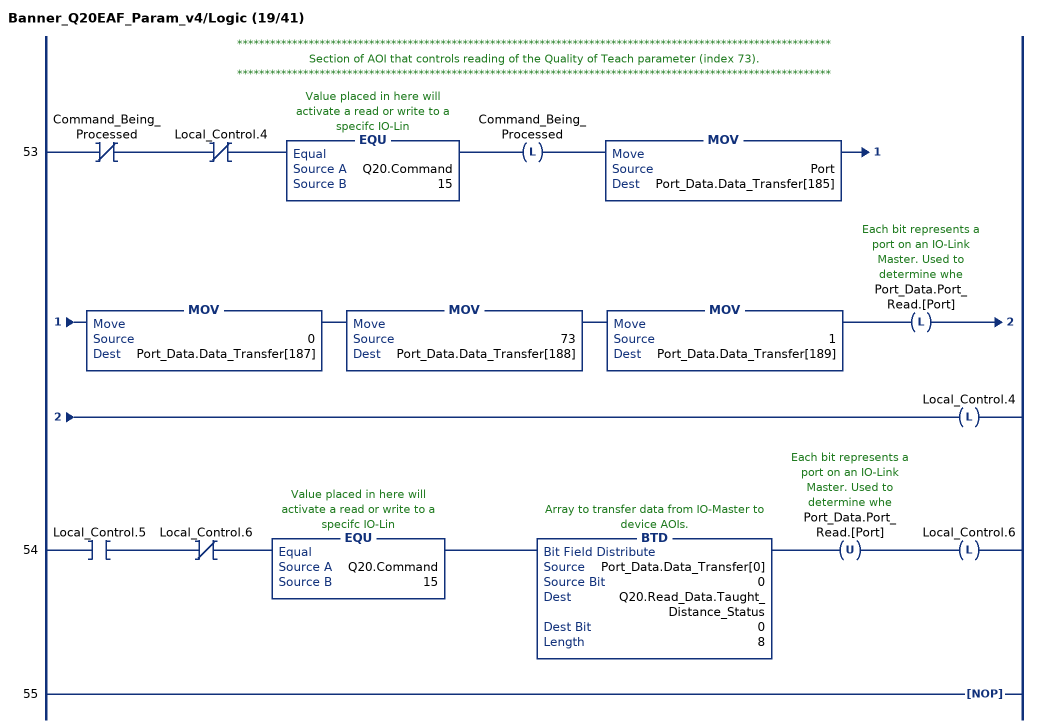
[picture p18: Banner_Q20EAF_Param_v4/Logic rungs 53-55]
   // ************************************************************************************************************
   // Section of AOI that controls reading of the Quality of Teach parameter (index 73).
   // ************************************************************************************************************
   53: XIO(Command_Being_Processed)XIO(Local_Control.4)EQU(Q20.Command,15)OTL(Command_Being_Processed)MOV(Port,Port_Data.Data_Transfer[185])MOV(0,Port_Data.Data_Transfer[187])MOV(73,Port_Data.Data_Transfer[188])MOV(1,Port_Data.Data_Transfer[189])OTL(Port_Data.Port_Read.[Port])OTL(Local_Control.4);
   54: XIC(Local_Control.5)XIO(Local_Control.6)EQU(Q20.Command,15)BTD(Port_Data.Data_Transfer[0],0,Q20.Read_Data.Taught_Distance_Status,0,8)OTU(Port_Data.Port_Read.[Port])OTL(Local_Control.6);
   55: NOP();
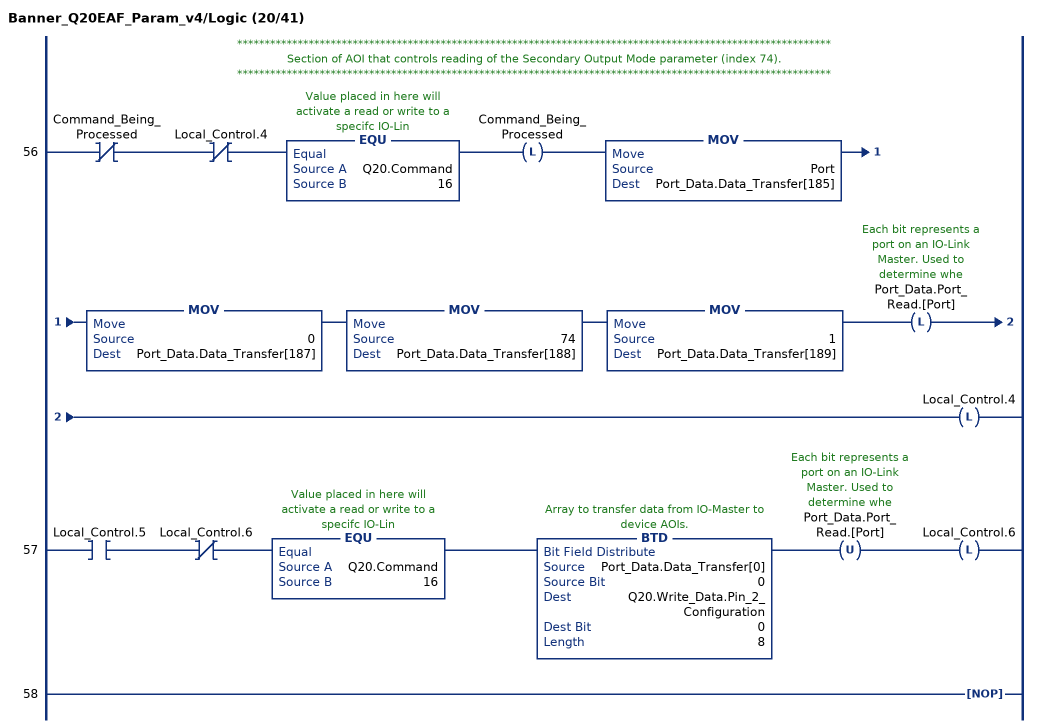
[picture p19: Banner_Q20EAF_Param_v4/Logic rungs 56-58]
   // ************************************************************************************************************
   // Section of AOI that controls reading of the Secondary Output Mode parameter (index 74).
   // ************************************************************************************************************
   56: XIO(Command_Being_Processed)XIO(Local_Control.4)EQU(Q20.Command,16)OTL(Command_Being_Processed)MOV(Port,Port_Data.Data_Transfer[185])MOV(0,Port_Data.Data_Transfer[187])MOV(74,Port_Data.Data_Transfer[188])MOV(1,Port_Data.Data_Transfer[189])OTL(Port_Data.Port_Read.[Port])OTL(Local_Control.4);
   57: XIC(Local_Control.5)XIO(Local_Control.6)EQU(Q20.Command,16)BTD(Port_Data.Data_Transfer[0],0,Q20.Write_Data.Pin_2_Configuration,0,8)OTU(Port_Data.Port_Read.[Port])OTL(Local_Control.6);
   58: NOP();
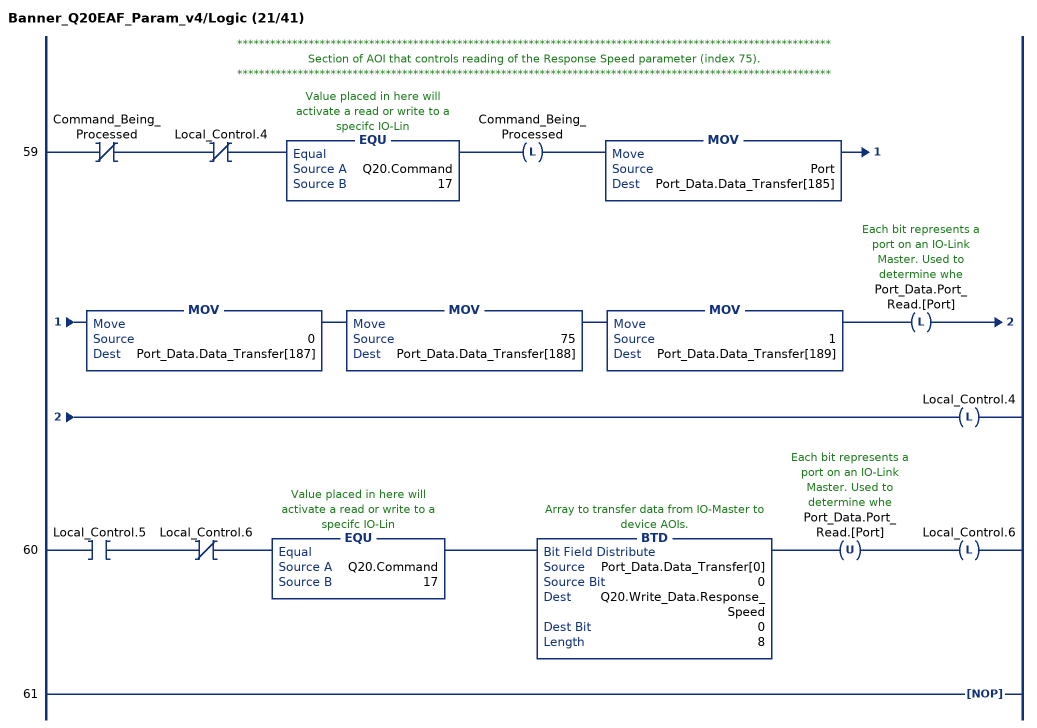
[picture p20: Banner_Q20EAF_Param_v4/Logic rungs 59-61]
   // ************************************************************************************************************
   // Section of AOI that controls reading of the Response Speed parameter (index 75).
   // ************************************************************************************************************
   59: XIO(Command_Being_Processed)XIO(Local_Control.4)EQU(Q20.Command,17)OTL(Command_Being_Processed)MOV(Port,Port_Data.Data_Transfer[185])MOV(0,Port_Data.Data_Transfer[187])MOV(75,Port_Data.Data_Transfer[188])MOV(1,Port_Data.Data_Transfer[189])OTL(Port_Data.Port_Read.[Port])OTL(Local_Control.4);
   60: XIC(Local_Control.5)XIO(Local_Control.6)EQU(Q20.Command,17)BTD(Port_Data.Data_Transfer[0],0,Q20.Write_Data.Response_Speed,0,8)OTU(Port_Data.Port_Read.[Port])OTL(Local_Control.6);
   61: NOP();
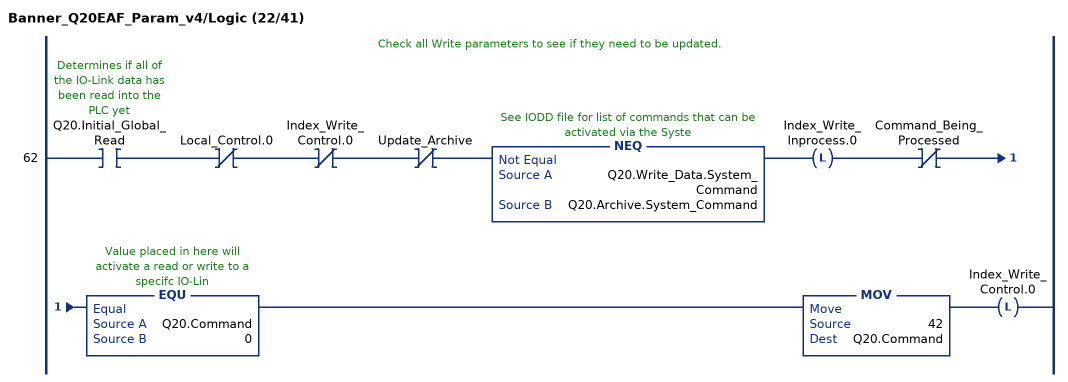
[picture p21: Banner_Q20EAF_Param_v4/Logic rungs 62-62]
   // Check all Write parameters to see if they need to be updated.
   62: XIC(Q20.Initial_Global_Read)XIO(Local_Control.0)XIO(Index_Write_Control.0)XIO(Update_Archive)NEQ(Q20.Write_Data.System_Command,Q20.Archive.System_Command)OTL(Index_Write_Inprocess.0)XIO(Command_Being_Processed)EQU(Q20.Command,0)MOV(42,Q20.Command)OTL(Index_Write_Control.0);
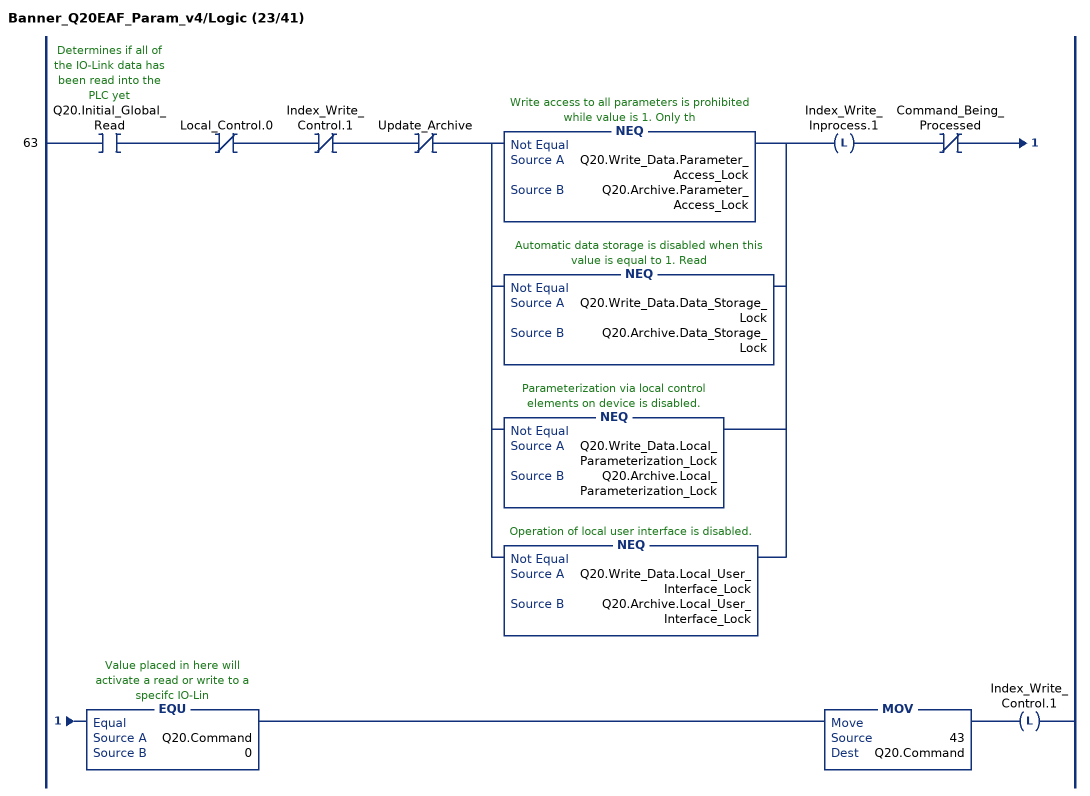
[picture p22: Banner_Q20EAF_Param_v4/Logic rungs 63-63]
   63: XIC(Q20.Initial_Global_Read)XIO(Local_Control.0)XIO(Index_Write_Control.1)XIO(Update_Archive)[NEQ(Q20.Write_Data.Parameter_Access_Lock,Q20.Archive.Parameter_Access_Lock) ,NEQ(Q20.Write_Data.Data_Storage_Lock,Q20.Archive.Data_Storage_Lock) ,NEQ(Q20.Write_Data.Local_Parameterization_Lock,Q20.Archive.Local_Parameterization_Lock) ,NEQ(Q20.Write_Data.Local_User_Interface_Lock,Q20.Archive.Local_User_Interface_Lock) ]OTL(Index_Write_Inprocess.1)XIO(Command_Being_Processed)EQU(Q20.Command,0)MOV(43,Q20.Command)OTL(Index_Write_Control.1);
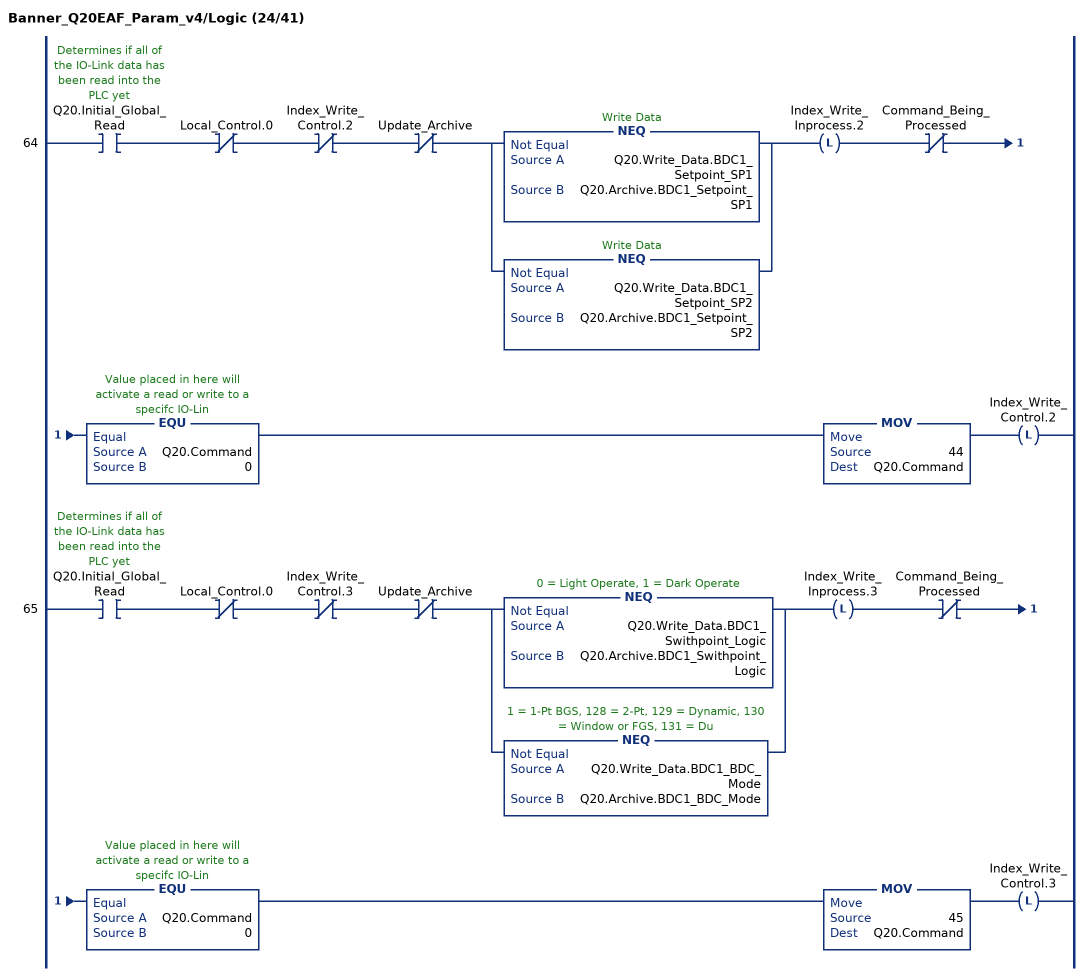
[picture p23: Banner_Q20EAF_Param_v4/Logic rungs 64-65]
   64: XIC(Q20.Initial_Global_Read)XIO(Local_Control.0)XIO(Index_Write_Control.2)XIO(Update_Archive)[NEQ(Q20.Write_Data.BDC1_Setpoint_SP1,Q20.Archive.BDC1_Setpoint_SP1) ,NEQ(Q20.Write_Data.BDC1_Setpoint_SP2,Q20.Archive.BDC1_Setpoint_SP2) ]OTL(Index_Write_Inprocess.2)XIO(Command_Being_Processed)EQU(Q20.Command,0)MOV(44,Q20.Command)OTL(Index_Write_Control.2);
   65: XIC(Q20.Initial_Global_Read)XIO(Local_Control.0)XIO(Index_Write_Control.3)XIO(Update_Archive)[NEQ(Q20.Write_Data.BDC1_Swithpoint_Logic,Q20.Archive.BDC1_Swithpoint_Logic) ,NEQ(Q20.Write_Data.BDC1_BDC_Mode,Q20.Archive.BDC1_BDC_Mode) ]OTL(Index_Write_Inprocess.3)XIO(Command_Being_Processed)EQU(Q20.Command,0)MOV(45,Q20.Command)OTL(Index_Write_Control.3);
